(* Logix 5000 Routine export MainRoutine; software revision 20.01 *)

TYPE RTA_STRING_4096 :   // string type; String Data Type with up to 4096 characters available
STRUCT
   LEN : DINT;
   DATA : SINT[4096];
END_STRUCT
END_TYPE

TYPE RTA_435NBX_490NBX :
STRUCT
   PLC_to_Gateway : RTA_STRING_4096;   // Contoller Scope Tag which must be defined in the 435NBX and 490NBX in the ASCII to PLC direction. This is the raw data from the ASCII device.
   Gateway_to_PLC : RTA_STRING_4096;   // Contoller Scope Tag which must be defined in the 435NBX and 490NBX in the PLC to ASCII direction. This is the raw data to send to the ASCII device.
   Data_to_Customer : RTA_STRING_4096;   // Contoller Scope Tag that the RTA_435NBX_490NBX_Gateway_to_PLC AOI uses to move the data to for the Customer to process.
   Data_from_Customer : RTA_STRING_4096;   // Contoller Scope Tag that the RTA_435NBX_490NBX_Gateway_to_PLC AOI uses to move the Customer's data in the PLC to the Tag the Gateway is monitoring.
   Active : INT;   // Contoller Scope Tag that the RTA_435NBX_490NBX_Heartbeat AOI uses to let the PLC know that the 435NBX / 490NBX is present and actively communicating to the PLC.
   Heartbeat : INT;   // Contoller Scope Tag that the 435NBX / 490NBX updates to let the PLC know the 435NBX / 490NBX is present and actively communicating.
END_STRUCT
END_TYPE

ADD_ON_INSTRUCTION RTA_435NBX_490NBX_Gateway_to_PLC   (* revision 1.0, vendor Real Time Automation, Inc. *)
// RTA's 435NBX / 490NBX Gateway to PLC handshaking
VAR_IN_OUT
   DataIn : RTA_STRING_4096; {required}
   DataOut : RTA_STRING_4096; {required}
END_VAR
VAR
   DataFromGateway : RTA_STRING_4096; {access None}
   DataToCustomer : RTA_STRING_4096; {access None}
END_VAR

ROUTINE Logic   (* ladder *)
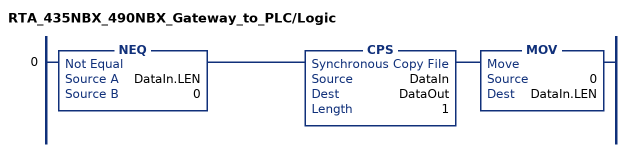
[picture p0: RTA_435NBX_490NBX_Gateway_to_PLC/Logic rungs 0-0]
   0: NEQ(DataIn.LEN,0)CPS(DataIn,DataOut,1)MOV(0,DataIn.LEN);
END_ROUTINE
END_ADD_ON_INSTRUCTION

ADD_ON_INSTRUCTION RTA_435NBX_490NBX_Heartbeat   (* revision 1.0, vendor Real Time Automation, Inc. *)
// RTA's 435NBX / 490NBX Heartbeat Handshaking
VAR_IN_OUT
   DataIn : INT; {required}
   DataOut : INT; {required}
END_VAR
VAR
   Previous_Value : INT; {access None}
   Number_of_Times_Inactive : INT; {access None}
END_VAR

ROUTINE Logic   (* ladder *)
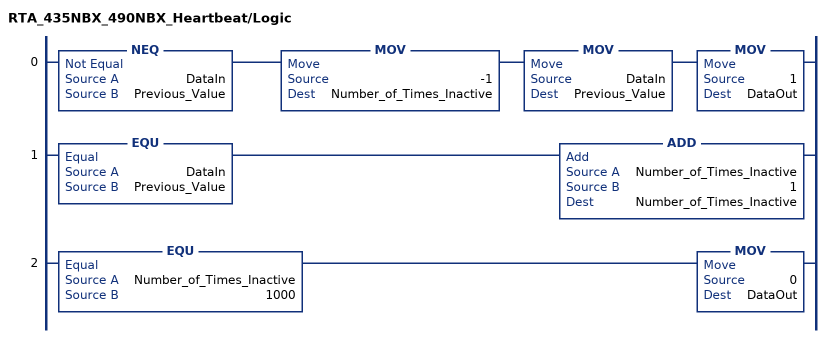
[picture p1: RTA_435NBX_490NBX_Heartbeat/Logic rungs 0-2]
   0: NEQ(DataIn,Previous_Value)MOV(-1,Number_of_Times_Inactive)MOV(DataIn,Previous_Value)MOV(1,DataOut);
   1: EQU(DataIn,Previous_Value)ADD(Number_of_Times_Inactive,1,Number_of_Times_Inactive);
   2: EQU(Number_of_Times_Inactive,1000)MOV(0,DataOut);
END_ROUTINE
END_ADD_ON_INSTRUCTION

ADD_ON_INSTRUCTION RTA_435NBX_490NBX_PLC_to_Gateway   (* revision 1.0, vendor Real Time Automation, Inc. *)
// RTA's 435NBX / 490NBX PLC to Gateway handshaking
VAR_IN_OUT
   DataIn : RTA_STRING_4096; {required}
   DataOut : RTA_STRING_4096; {required}
END_VAR
VAR
   DataToGateway : RTA_STRING_4096; {access None}
   DataFromCustomer : RTA_STRING_4096; {access None}
   NULL_Tag : RTA_STRING_4096; {access None}
END_VAR

ROUTINE Logic   (* ladder *)
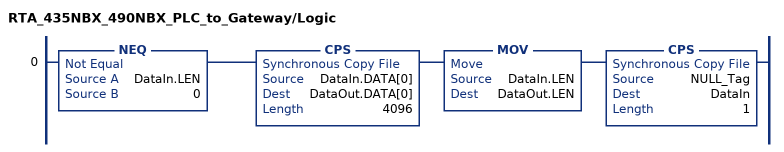
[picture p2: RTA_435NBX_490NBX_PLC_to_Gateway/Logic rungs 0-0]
   0: NEQ(DataIn.LEN,0)CPS(DataIn.DATA[0],DataOut.DATA[0],4096)MOV(DataIn.LEN,DataOut.LEN)CPS(NULL_Tag,DataIn,1);
END_ROUTINE
END_ADD_ON_INSTRUCTION

VAR_GLOBAL   (* controller tags *)
   RTA_435NBX_490NBX_Heartbeat : RTA_435NBX_490NBX_Heartbeat;
   RTA_435NBX_490NBX_PLC_to_Gateway : RTA_435NBX_490NBX_PLC_to_Gateway;   // RTA's 435NBX / 490NBX PLC to Gateway Handshaking
   RTA_435NBX_490NBX_Gateway_to_PLC : RTA_435NBX_490NBX_Gateway_to_PLC;
   RTA_435NBX_490NBX : RTA_435NBX_490NBX;
END_VAR

PROGRAM MainProgram

ROUTINE MainRoutine   (* ladder *)
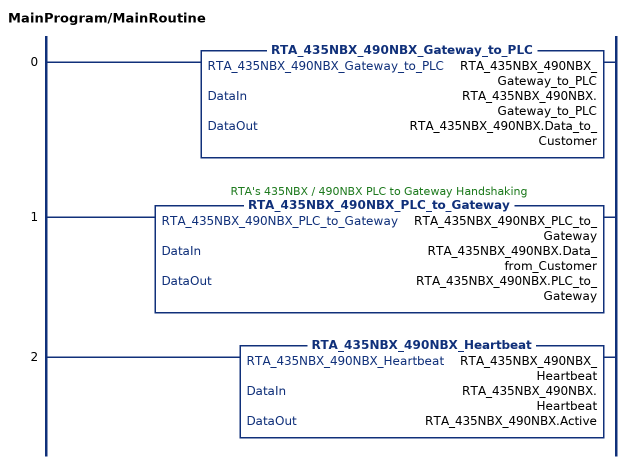
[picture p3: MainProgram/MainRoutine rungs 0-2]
   0: RTA_435NBX_490NBX_Gateway_to_PLC(RTA_435NBX_490NBX_Gateway_to_PLC,RTA_435NBX_490NBX.Gateway_to_PLC,RTA_435NBX_490NBX.Data_to_Customer);
   1: RTA_435NBX_490NBX_PLC_to_Gateway(RTA_435NBX_490NBX_PLC_to_Gateway,RTA_435NBX_490NBX.Data_from_Customer,RTA_435NBX_490NBX.PLC_to_Gateway);
   2: RTA_435NBX_490NBX_Heartbeat(RTA_435NBX_490NBX_Heartbeat,RTA_435NBX_490NBX.Heartbeat,RTA_435NBX_490NBX.Active);
END_ROUTINE
END_PROGRAM
